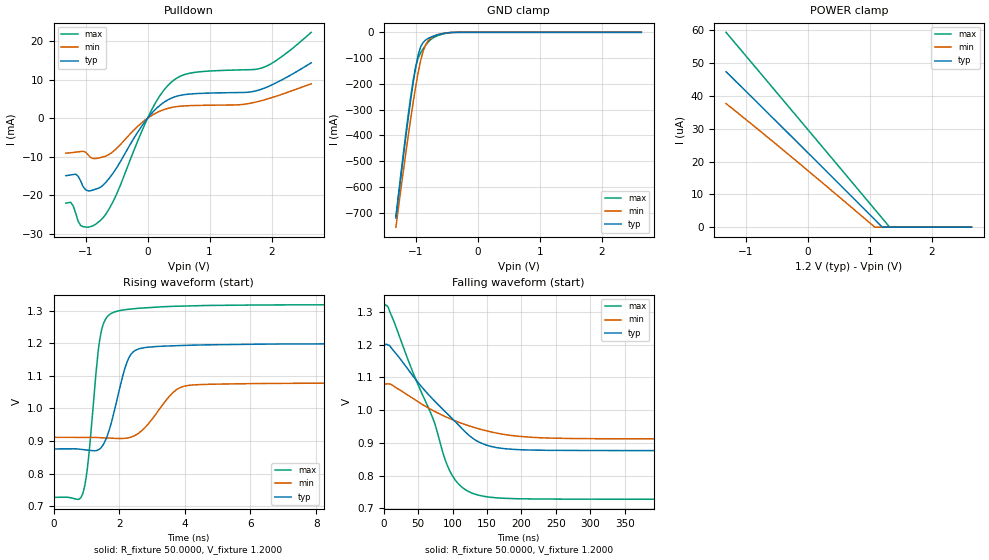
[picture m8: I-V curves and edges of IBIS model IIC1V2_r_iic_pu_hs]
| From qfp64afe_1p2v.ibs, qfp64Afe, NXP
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[Model] IIC1V2_r_iic_pu_hs
|   Model IIC1V2_r_iic_pu_hs
| This model was characterised for following simulation conditions:
| External (pad) voltage:
|   - Typ: 1.2V,   - Min: 1.08V,   - Max: 1.32V
| Library cells for typ/min/max conditions are connected as defined below:
|  IO - External Pad
|  A - Core Input
|  EN - Output Buffer Enable
|  BOOST - vdde
|  ECS - vdd
|  EGP - gnd
|  ENZI - vdd
|  EPD - vdd
|  EPUN - gnd
|  SSEL - vdd
|  ZI - NC
|  ZIF - NC
|  gnd - gnd
|  gnde - gnde
|  vdd - vdd
|  vdde - vdde
| All other pins connected to ground
Model_type I/O_open_drain
Polarity   Non-Inverting
Enable   Active-Low
Vinl =   0.5400V
Vinh =   1.2600V
Vmeas =  0.9000V
Cref =   0.0F
Rref =   1.0000k
Vref =   1.2000V
C_comp   3.6164pF   3.4768pF   3.7417pF
|C_comp_pullup   0.9402pF   0.8991pF   0.9548pF
|C_comp_pulldown   2.3240pF   2.4771pF   2.1787pF
[Model Spec]
| variable   typ   min   max
Vinh   0.3600V   0.3240V   0.3960V
Vinl   0.8400V   0.7560V   0.9240V
Vmeas   0.6000V   0.5400V   0.6600V
Vref   1.2000V   1.0800V   1.3200V
Cref   0.0F   0.0F   0.0F
Rref   1.0000k   1.0000k   1.0000k
[Temperature Range]   25.0000   0.1250k   -40.0000
[Voltage Range]   1.2000V   1.0800V   1.3200V
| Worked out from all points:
|   slope of the pulldown table from 0 to 0.18 V, typ, clamps not added: 58.3 ohm
|   GND clamp passes 1 mA (typ) near -0.45 V on its own axis
|   rising waveform, R_fixture 50.0000, V_fixture 1.2000: 20-80 % time 495ps typ, 789ps min, 329ps max; typ from 0.876 V to 1.2 V
|   falling waveform, R_fixture 50.0000, V_fixture 1.2000: 20-80 % time 83.2ns typ, 99.1ns min, 62.6ns max; typ from 1.2 V to 0.876 V
[Pulldown]
|Voltage   I(typ)   I(min)   I(max)
-1.32V    -14.96mA   -9.099mA   -22.09mA
-1.24V    -14.75mA   -8.982mA   -21.89mA
-1.16V    -14.56mA   -8.83mA    -24.7mA
-1.04V    -17.82mA   -8.609mA   -28.21mA
-920mV    -18.88mA   -10.21mA   -28.21mA
-720mV    -17.44mA   -10.07mA   -25.94mA
-520mV    -13.41mA   -8.157mA   -20.44mA
80mV      1.521mA    840uA      2.628mA
440mV     5.569mA    2.951mA    10.1mA
760mV     6.377mA    3.307mA    11.92mA
1.84V     7.555mA    4.581mA    13.06mA
2.64V     14.41mA    8.944mA    22.34mA
[GND_clamp]
|Voltage   I(typ)   I(min)   I(max)
-1.32V    -720.7mA   -756.5mA   -713.8mA
-1.12V    -330.9mA   -399.5mA   -316.8mA
-1.04V    -192.4mA   -269.2mA   -184.4mA
-1V       -133.6mA   -209.3mA   -133.5mA
-960mV    -86.74mA   -154.7mA   -99.46mA
-920mV    -55.69mA   -108.2mA   -79.02mA
-880mV    -39.02mA   -72.35mA   -63.71mA
-840mV    -29.9mA    -48mA      -50.26mA
-760mV    -18.93mA   -23.39mA   -28.32mA
-640mV    -9.22mA    -8.628mA   -12.73mA
-400mV    -335.3uA   -402.3uA   -442.6uA
2.64V     0A         0A         0A
[POWER_clamp]
|Voltage   I(typ)   I(min)   I(max)
-1.32V    47.4uA     37.67uA    59.39uA
-280mV    27.94uA    21.65uA    36.04uA
1.08V     2.274uA    0A         5.413uA
1.2V      0A         0A         2.707uA
1.32V     0A         0A         0A
2.64V     0A         0A         0A
[Ramp]
| variable   typ   min   max
dV/dt_r  0.1940/0.4950n   0.1007/0.7892n   0.3552/0.3288n
dV/dt_f  0.1940/83.2200n   0.1007/98.9601n   0.3551/62.5787n
R_load = 50.0000
[Rising Waveform]
R_fixture= 50.0000
V_fixture= 1.2000
V_fixture_min= 1.0800
V_fixture_max= 1.3200
|time   V(typ)   V(min)   V(max)
0s        875.8mV    911.4mV    727.2mV
905ps     873.9mV    911.7mV    743.7mV
1.065ns   871.8mV    911.6mV    846.3mV
1.401ns   875.3mV    910.5mV    1.207V
1.677ns   927.8mV    909.1mV    1.286V
2.172ns   1.123V     908.3mV    1.303V
2.475ns   1.177V     916.9mV    1.306V
3.882ns   1.193V     1.065V     1.314V
6.019ns   1.197V     1.076V     1.317V
1us       1.199V     1.079V     1.319V
[Falling Waveform]
R_fixture= 50.0000
V_fixture= 1.2000
V_fixture_min= 1.0800
V_fixture_max= 1.3200
|time   V(typ)   V(min)   V(max)
0s        1.199V     1.079V     1.319V
6.599ns   1.199V     1.08V      1.314V
41.29ns   1.108V     1.037V     1.121V
69.63ns   1.037V     1.001V     984.6mV
95.58ns   982.4mV    974.3mV    815.7mV
113.7ns   943.4mV    959.2mV    764.2mV
137ns     903.7mV    943.2mV    740.2mV
173ns     882.6mV    926.1mV    730.5mV
258ns     876.7mV    913.6mV    727.8mV
1us       875.9mV    911.5mV    727.2mV
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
